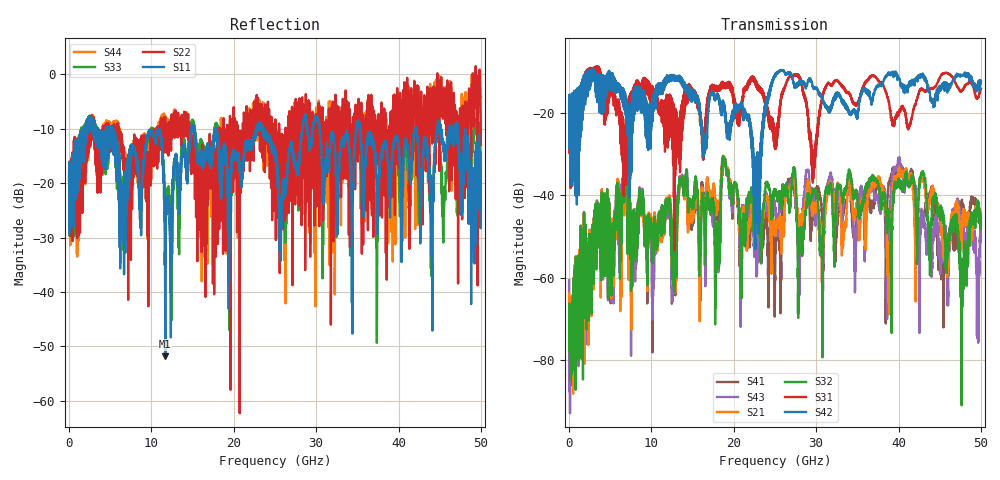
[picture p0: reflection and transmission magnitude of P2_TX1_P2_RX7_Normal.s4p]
!Keysight Technologies,N5225B,MY57041031,A.13.20.10
!Date: Friday, May 31, 2019 11:37:29
!Correction: S11(Full 4 Port(1,2,3,4))
!S12(Full 4 Port(1,2,3,4))
!S13(Full 4 Port(1,2,3,4))
!S14(Full 4 Port(1,2,3,4))
!S21(Full 4 Port(1,2,3,4))
!S22(Full 4 Port(1,2,3,4))
!S23(Full 4 Port(1,2,3,4))
!S24(Full 4 Port(1,2,3,4))
!S31(Full 4 Port(1,2,3,4))
!S32(Full 4 Port(1,2,3,4))
!S33(Full 4 Port(1,2,3,4))
!S34(Full 4 Port(1,2,3,4))
!S41(Full 4 Port(1,2,3,4))
!S42(Full 4 Port(1,2,3,4))
!S43(Full 4 Port(1,2,3,4))
!S44(Full 4 Port(1,2,3,4))
!S4P File: Measurements: <S11,S12,S13,S14>,
!<S21,S22,S23,S24>,
!<S31,S32,S33,S34>,
!<S41,S42,S43,S44>:
# Hz S  dB  R 50.0
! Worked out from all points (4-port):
!   5000 points, 10 MHz to 50 GHz, reference 50 ohm
!   strongest paths, dB at 10 MHz, 12.51 GHz, 25.01 GHz, 37.51 GHz, 50 GHz:
!     S42: -19.5, -11.9, -11.4, -13.3, -12.3
!     S31: -19.4, -17.3, -28.8, -12.1, -14.2
!     S32: -77.6, -51.0, -39.6, -37.2, -47.1
!     S21: -63.6, -52.7, -49.7, -35.7, -46.5
!     S43: -60.6, -53.5, -43.5, -40.4, -48.1
!     S41: -65.1, -56.5, -59.5, -37.2, -46.5
!   lowest |S11| = -51.8 dB at 11.69 GHz (marker M1), VSWR 1.01, Z = 49.8 - j0.164 ohm
!   |S11| at or under -10 dB: 5.36 GHz to 10.81 GHz (5.449 GHz wide, 67.4 % of centre); 17.89 GHz to 22.7 GHz (4.805 GHz wide, 23.7 % of centre); 35.31 GHz to 41.96 GHz (6.643 GHz wide, 17.2 % of centre)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
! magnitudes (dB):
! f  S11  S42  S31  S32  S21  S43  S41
! 10 MHz  -19.6  -19.5  -19.4  -77.6  -63.6  -60.6  -65.1
! 6.83 GHz  -32.8  -18.9  -30.6  -34.2  -36.4  -32.7  -34.2
! 11.69 GHz  -51.8  -12.6  -22.9  -44.3  -44.7  -44.7  -44.5
! 18.88 GHz  -12.9  -19.8  -13.1  -31.3  -31.1  -31.5  -31.0
! 22.81 GHz  -9.7  -36.2  -14.0  -46.3  -43.6  -59.2  -45.9
! 25.62 GHz  -28.0  -9.7  -19.1  -41.2  -47.3  -42.8  -55.0
! 50 GHz  -17.3  -12.3  -14.2  -47.1  -46.5  -48.1  -46.5
